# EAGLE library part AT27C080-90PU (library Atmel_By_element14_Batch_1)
8-Megabit (1M x 8) OTP EPROM
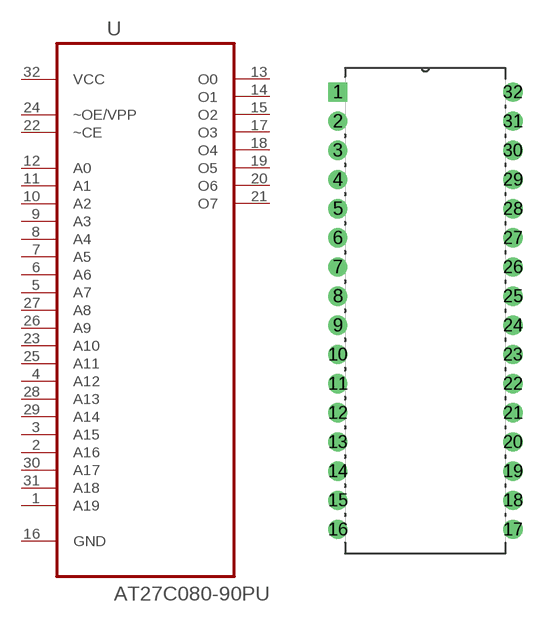
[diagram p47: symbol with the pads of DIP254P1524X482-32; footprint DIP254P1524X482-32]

Designator prefix U

## AT27C080-90PU (MPN: AT27C080-90PU; OC_FARNELL: 1455026; OC_NEWARK: 58M3824; PACKAGE: PDIP-32; SUPPLIER: Atmel)  [DIP254P1524X482-32]
1  A19  in
2  A16  in
3  A15  in
4  A12  in
5  A7  in
6  A6  in
7  A5  in
8  A4  in
9  A3  in
10  A2  in
11  A1  in
12  A0  in
13  O0  out
14  O1  out
15  O2  out
16  GND  out
17  O3  out
18  O4  out
19  O5  out
20  O6  out
21  O7  out
22  ~CE  in
23  A10  in
24  ~OE/VPP  in
25  A11  in
26  A9  in
27  A8  in
28  A13  in
29  A14  in
30  A17  in
31  A18  in
32  VCC  pwr

## Footprint DIP254P1524X482-32 (pad centres in mm)
drill 1.118 square: 1 -15.24,38.1
drill 1.118: 2 -15.24,35.56; 3 -15.24,33.02; 4 -15.24,30.48; 5 -15.24,27.94; 6 -15.24,25.4; 7 -15.24,22.86; 8 -15.24,20.32; 9 -15.24,17.78; 10 -15.24,15.24; 11 -15.24,12.7; 12 -15.24,10.16; 13 -15.24,7.62; 14 -15.24,5.08; 15 -15.24,2.54; 16 -15.24,0; 17 0,0; 18 0,2.54; 19 0,5.08; 20 0,7.62; 21 0,10.16; 22 0,12.7; 23 0,15.24; 24 0,17.78; 25 0,20.32; 26 0,22.86; 27 0,25.4; 28 0,27.94; 29 0,30.48; 30 0,33.02; 31 0,35.56; 32 0,38.1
